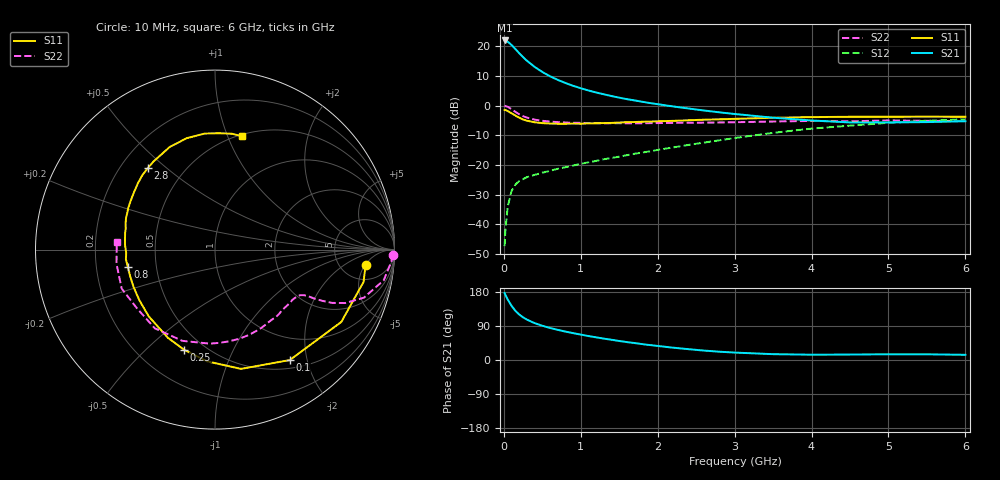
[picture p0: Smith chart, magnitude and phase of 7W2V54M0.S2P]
! Infineon Technologies  Discrete & RF Semiconductors
! BFS17W
! Si NPN RF Bipolar Junction Transistor in SOT323
! VCE = 2.5 V  IC = 4 mA
! Common Emitter S-Parameters:  August  1999
# GHz  S  MA  R  50
!  f  S11  S21  S12  S22
! GHz  MAG  ANG  MAG  ANG  MAG  ANG  MAG  ANG
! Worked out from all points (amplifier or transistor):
!   36 points, 10 MHz to 6 GHz, reference 50 ohm
!   highest |S21| = 21.9 dB at 10 MHz (marker M1)
!   |S21| within 3 dB of that: start of sweep to 153.9 MHz
!   unconditionally stable (mu >= 1): 596.5 MHz to 3.265 GHz; 4 GHz to end of sweep
!   at 250 MHz: K = 0.53, MSG = 20.5 dB, |S12| = -24.7 dB
!   at 1.4 GHz: K = 1.29, MAG = 7.2 dB, |S12| = -17.6 dB
!   at 6 GHz: K = 1.10, MAG = -2.2 dB, |S12| = -4.6 dB
!   S11 on the Smith chart (normalised r, x): 10 MHz: 9, -5; 100 MHz: 0.62, -1.71; 250 MHz: 0.39, -0.66; 800 MHz: 0.34, -0.09; 2.8 GHz: 0.31, +0.43; 6 GHz: 0.52, +1.13
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0.01  0.8434 -6.0  12.51 176.5  0.0043 81.8  0.9946 -1.7
0.02  0.847 -12.3  12.47 171.8  0.008 85.0  0.9828 -4.3
0.05  0.811 -29.8  11.94 159.8  0.0198 75.9  0.9554 -10.3
0.1  0.7432 -55.9  10.5 143.1  0.0366 63.3  0.8716 -17.9
0.15  0.6802 -77.7  8.964 129.8  0.0468 54.4  0.7844 -22.3
0.2  0.624 -94.1  7.642 120.1  0.0538 50.6  0.716 -24.5
0.25  0.5838 -107.2  6.545 112.6  0.0579 47.0  0.6639 -25.5
0.3  0.5571 -118.1  5.697 106.6  0.0625 45.9  0.629 -26.1
0.4  0.5241 -134.7  4.491 97.3  0.0683 45.2  0.5804 -26.6
0.5  0.5073 -146.2  3.688 90.4  0.0742 46.2  0.5553 -27.2
0.6  0.4991 -155.2  3.118 84.5  0.0798 47.7  0.5385 -28.1
0.8  0.495 -168.6  2.404 75.0  0.0918 51.1  0.5195 -31.4
0.9  0.4993 -173.7  2.157 70.9  0.0977 52.5  0.5139 -33.1
1.1  0.5018 177.2  1.798 63.2  0.111 54.8  0.5086 -37.6
1.3  0.5091 169.6  1.551 56.4  0.125 57.0  0.5038 -42.7
1.6  0.5264 160.3  1.285 47.3  0.1463 59.4  0.5028 -50.6
2.2  0.554 144.3  0.969 32.5  0.1978 62.5  0.5117 -68.2
2.8  0.5881 129.7  0.772 21.9  0.2603 62.0  0.5201 -87.2
3.5  0.6248 113.9  0.626 15.4  0.3481 57.6  0.5399 -109.7
4.5  0.649 95.0  0.521 14.4  0.4598 45.8  0.5441 -143.2
5.5  0.6523 81.6  0.528 15.0  0.5534 33.5  0.5547 -171.8
6  0.6489 76.4  0.546 13.7  0.5897 27.6  0.5487 175.7
